(* Logix 5000 AddOnInstructionDefinition export AMCI_ANG1E_Home_CCW; software revision 20.03 *)

ADD_ON_INSTRUCTION AMCI_ANG1E_Home_CCW   (* revision 5.0, vendor AMCI, ExecuteEnableInFalse *)
// Revision note:
// Version 5.0 added the (hidden) ability to program the motor current and unlatched the error bit if the rung goes false.
VAR_INPUT
   Axis_Status_Bits : INT; {required}
   slot_axis_number : INT; {required}
   Type_0_for_standard_1_for_indexed : BOOL;
   Programmed_Speed : DINT; {required}
   Acceleration : INT; {required}
   Deceleration : INT; {required}
   motor_current : INT;
   jerk : INT;
END_VAR
VAR_IN_OUT
   AMCI_ANG1E_output_data : INT[10]; {required}
END_VAR
VAR_OUTPUT
   EN : BOOL; {access Read Only, visible}
   ER : BOOL; {access Read Only, visible}
END_VAR
VAR
   Upper_Result_X_1000 : DINT;
   command_data_block : INT[10];
        [0]   // Command Bits MSW
        [1]   // Command Bits LSW
        [2]   // Upper Target Position
        [3]   // Lower Target Position
        [4]   // Upper Programmed Speed
        [5]   // Lower Programmed Speed
   index : INT;
END_VAR

ROUTINE EnableInFalse   (* ladder *)
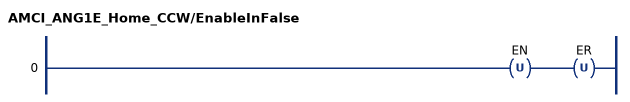
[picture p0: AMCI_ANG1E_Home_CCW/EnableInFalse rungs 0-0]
   0: OTU(EN)OTU(ER);
END_ROUTINE

ROUTINE Logic   (* ladder *)
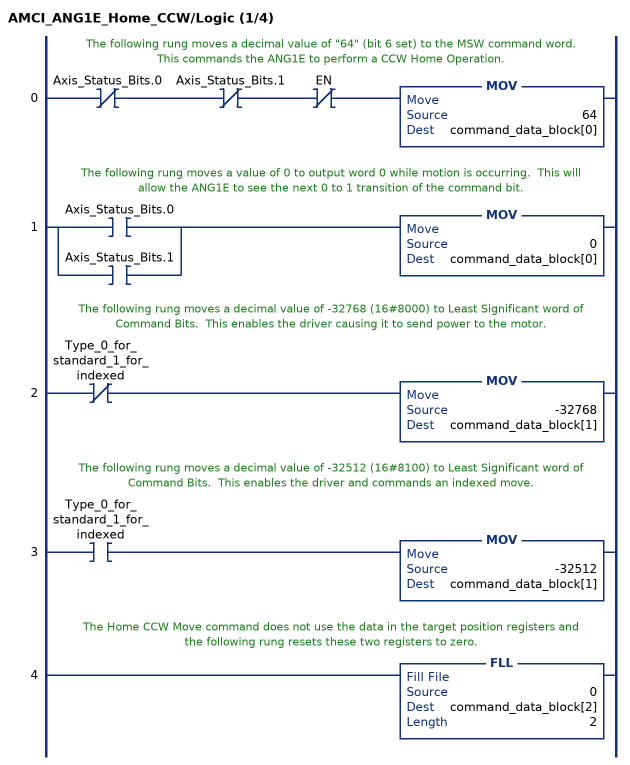
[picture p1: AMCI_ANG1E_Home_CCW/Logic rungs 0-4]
   // The following rung moves a decimal value of "64" (bit 6 set) to the MSW command word.  This commands the ANG1E to perform a CCW Home Operation.
   0: XIO(Axis_Status_Bits.0)XIO(Axis_Status_Bits.1)XIO(EN)MOV(64,command_data_block[0]);
   // The following rung moves a value of 0 to output word 0 while motion is occurring.  This will allow the ANG1E to see the next 0 to 1 transition of the command bit.
   1: [XIC(Axis_Status_Bits.0) ,XIC(Axis_Status_Bits.1) ]MOV(0,command_data_block[0]);
   // The following rung moves a decimal value of -32768 (16#8000) to Least Significant word of Command Bits.  This enables the driver causing it to send power to the motor.
   2: XIO(Type_0_for_standard_1_for_indexed)MOV(-32768,command_data_block[1]);
   // The following rung moves a decimal value of -32512 (16#8100) to Least Significant word of Command Bits.  This enables the driver and commands an indexed move.
   3: XIC(Type_0_for_standard_1_for_indexed)MOV(-32512,command_data_block[1]);
   // The Home CCW Move command does not use the data in the target position registers and the following rung resets these two registers to zero.
   4: FLL(0,command_data_block[2],2);
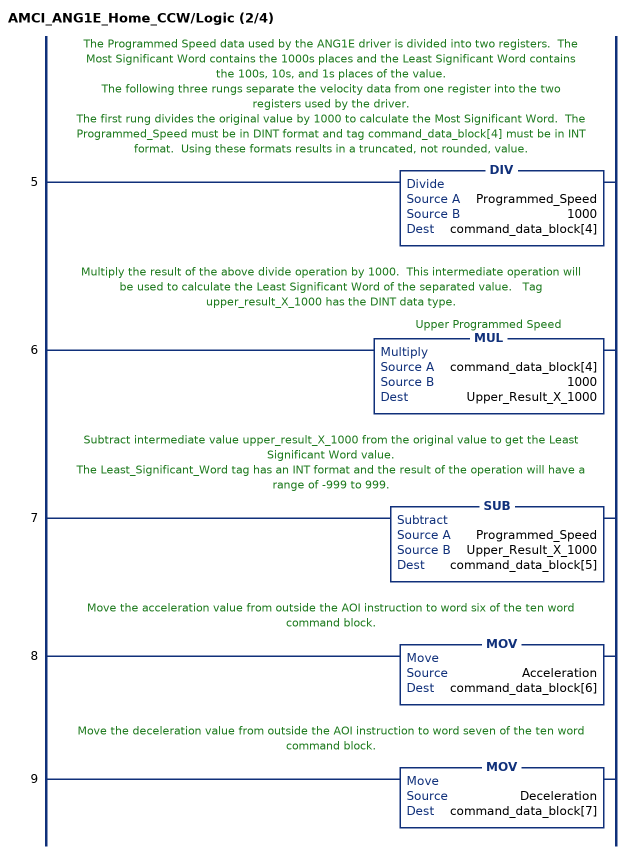
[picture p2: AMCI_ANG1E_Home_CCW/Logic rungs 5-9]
   // The Programmed Speed data used by the ANG1E driver is divided into two registers.  The Most Significant Word contains the 1000s places and the Least Significant Word contains the 100s, 10s, and 1s places of the value.
   // The following three rungs separate the velocity data from one register into the two registers used by the driver.
   // The first rung divides the original value by 1000 to calculate the Most Significant Word.  The Programmed_Speed must be in DINT format and tag command_data_block[4] must be in INT format.  Using these formats results in a truncated, not rounded, value.
   5: DIV(Programmed_Speed,1000,command_data_block[4]);
   // Multiply the result of the above divide operation by 1000.  This intermediate operation will be used to calculate the Least Significant Word of the separated value.   Tag upper_result_X_1000 has the DINT data type.
   6: MUL(command_data_block[4],1000,Upper_Result_X_1000);
   // Subtract intermediate value upper_result_X_1000 from the original value to get the Least Significant Word value.
   // The Least_Significant_Word tag has an INT format and the result of the operation will have a range of -999 to 999.
   7: SUB(Programmed_Speed,Upper_Result_X_1000,command_data_block[5]);
   // Move the acceleration value from outside the AOI instruction to word six of the ten word command block.
   8: MOV(Acceleration,command_data_block[6]);
   // Move the deceleration value from outside the AOI instruction to word seven of the ten word command block.
   9: MOV(Deceleration,command_data_block[7]);
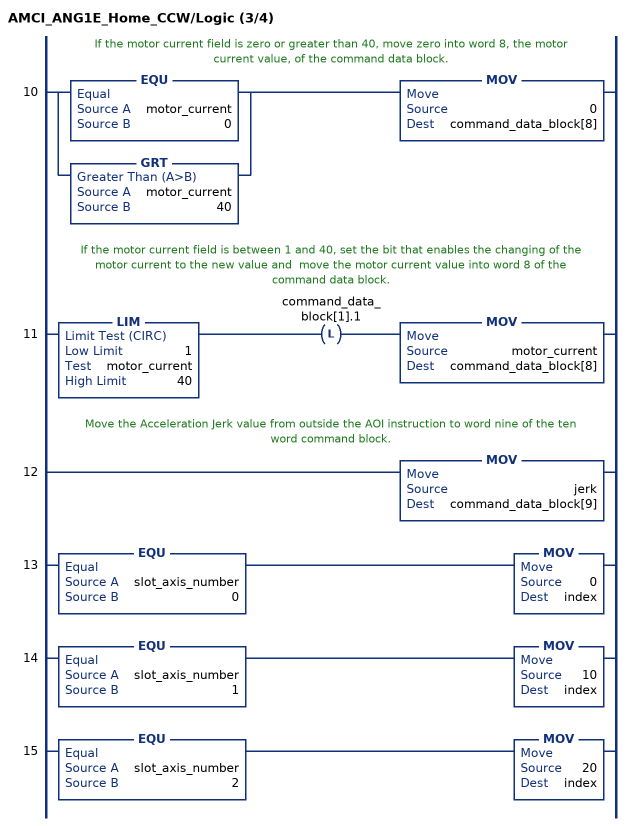
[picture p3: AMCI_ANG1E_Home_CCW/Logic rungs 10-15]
   // If the motor current field is zero or greater than 40, move zero into word 8, the motor current value, of the command data block.
   10: [EQU(motor_current,0) ,GRT(motor_current,40) ]MOV(0,command_data_block[8]);
   // If the motor current field is between 1 and 40, set the bit that enables the changing of the motor current to the new value and  move the motor current value into word 8 of the command data block.
   11: LIM(1,motor_current,40)OTL(command_data_block[1].1)MOV(motor_current,command_data_block[8]);
   // Move the Acceleration Jerk value from outside the AOI instruction to word nine of the ten word command block.
   12: MOV(jerk,command_data_block[9]);
   13: EQU(slot_axis_number,0)MOV(0,index);
   14: EQU(slot_axis_number,1)MOV(10,index);
   15: EQU(slot_axis_number,2)MOV(20,index);
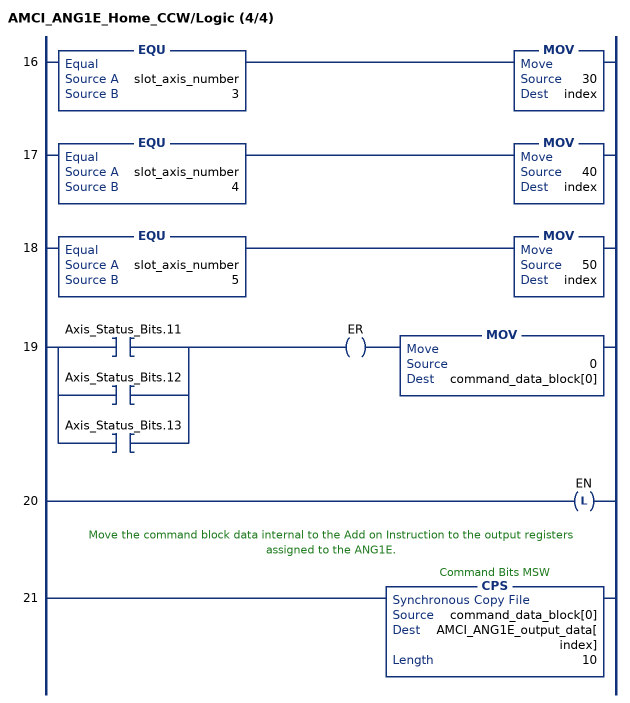
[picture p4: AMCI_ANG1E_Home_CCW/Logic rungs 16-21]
   16: EQU(slot_axis_number,3)MOV(30,index);
   17: EQU(slot_axis_number,4)MOV(40,index);
   18: EQU(slot_axis_number,5)MOV(50,index);
   19: [XIC(Axis_Status_Bits.11) ,XIC(Axis_Status_Bits.12) ,XIC(Axis_Status_Bits.13) ]OTE(ER)MOV(0,command_data_block[0]);
   20: OTL(EN);
   // Move the command block data internal to the Add on Instruction to the output registers assigned to the ANG1E.
   21: CPS(command_data_block[0],AMCI_ANG1E_output_data[index],10);
END_ROUTINE
END_ADD_ON_INSTRUCTION
